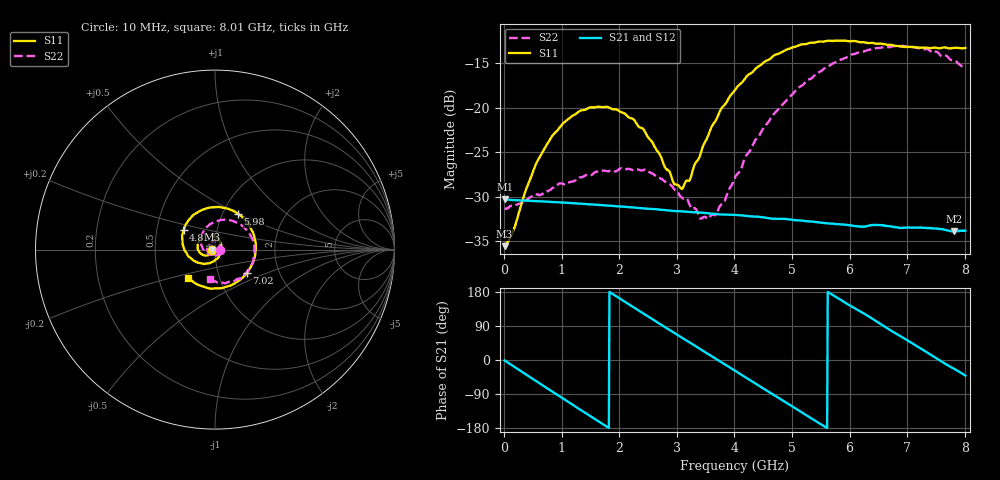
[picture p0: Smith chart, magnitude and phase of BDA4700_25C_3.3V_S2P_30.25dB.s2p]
!Agilent Technologies,E5071B,MY42404982,A.09.10
!Date: Mon Oct 20 18:15:48 2025
!Data & Calibration Information:
!Freq	S11:SOLT2(ON)	S21:SOLT2(ON)	S12:SOLT2(ON)	S22:SOLT2(ON)
# Hz S RI R 50
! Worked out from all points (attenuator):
!   801 points, 10 MHz to 8.01 GHz, reference 50 ohm
!   highest |S21| = -30.29 dB at 20 MHz (marker M1); lowest = -33.9 dB at 7.81 GHz (marker M2)
!   lowest |S11| = -35.5 dB at 10 MHz (marker M3), VSWR 1.03, Z = 48.4 - j0.0993 ohm
!   |S11| at or under -10 dB: start of sweep to end of sweep
!   |S22| runs from -32.5 to -13.0 dB; largest |S21 - S12| = 0.00041
!   S11 on the Smith chart (normalised r, x): 10 MHz: 0.97, -0.00; 4.82 GHz: 0.69, +0.15; 5.98 GHz: 1.18, +0.50; 7.02 GHz: 1.37, -0.38; 8.01 GHz: 0.71, -0.24
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1e7  -0.0167 -0.00103  0.0306 -0.000623  0.0306 -0.000669  0.0271 -0.000806
2e7  -0.017 -0.00172  0.0306 -0.00116  0.0306 -0.00119  0.0271 -0.00107
7e8  -0.0487 -0.0332  0.0103 -0.0279  0.0103 -0.0279  0.00615 -0.033
1.03e9  -0.0788 -0.0231  -0.00621 -0.0287  -0.00621 -0.0287  -0.0163 -0.0336
1.35e9  -0.0968 0.00609  -0.0199 -0.0209  -0.0199 -0.021  -0.0364 -0.0182
2.08e9  -0.0515 0.0781  -0.0253 0.0116  -0.0253 0.0116  -0.0302 0.0336
2.68e9  0.0239 0.0508  -0.00358 0.0266  -0.00363 0.0266  0.0127 0.0383
2.95e9  0.0355 0.0121  0.0081 0.0251  0.00809 0.025  0.0256 0.024
3.1e9  0.0332 -0.0119  0.014 0.0221  0.0138 0.0222  0.0287 0.0119
3.23e9  0.0253 -0.0305  0.0181 0.0186  0.0182 0.0185  0.028 0.00298
3.55e9  -0.0155 -0.0689  0.0246 0.00671  0.0247 0.00664  0.0131 -0.02
3.69e9  -0.0409 -0.0764  0.0253 0.000865  0.0253 0.000793  0.00169 -0.0252
4.01e9  -0.1063 -0.0676  0.0221 -0.0118  0.022 -0.0118  -0.0309 -0.026
4.36e9  -0.1645 -0.0108  0.0117 -0.0215  0.0117 -0.0216  -0.0657 0.00115
4.82e9  -0.175 0.1078  -0.00622 -0.023  -0.00602 -0.023  -0.0769 0.069
5.35e9  -0.071 0.2212  -0.0209 -0.00955  -0.0208 -0.00971  -0.016 0.1465
5.98e9  0.1285 0.1992  -0.0182 0.0123  -0.0183 0.0122  0.1258 0.1489
6.68e9  0.2254 -0.0159  0.00331 0.0214  0.00339 0.0214  0.2195 0.000645
7.02e9  0.1781 -0.1299  0.0136 0.0164  0.0136 0.0163  0.2003 -0.0901
7.45e9  0.0448 -0.2132  0.0207 0.00361  0.0207 0.00356  0.1135 -0.1702
7.81e9  -0.0873 -0.1988  0.0186 -0.00787  0.0187 -0.00788  0.0178 -0.1839
8.01e9  -0.148 -0.1589  0.0154 -0.0134  0.0154 -0.0134  -0.0296 -0.1636
